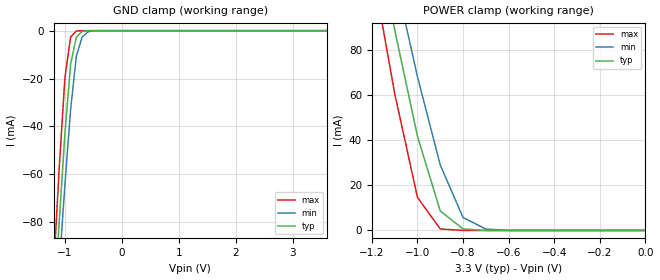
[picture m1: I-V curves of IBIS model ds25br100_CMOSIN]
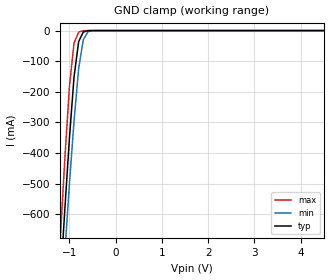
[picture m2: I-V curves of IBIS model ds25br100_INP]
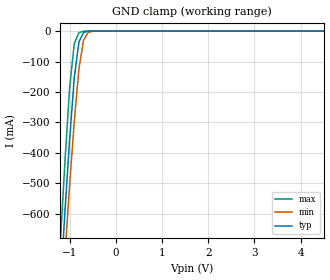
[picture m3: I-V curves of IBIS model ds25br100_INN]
|   National Semiconductor Corporation
|   IBIS Model
|   of
|   ds25br100
|  (no equalization, no pre-emphasis)
[IBIS Ver]   3.2
[Comment Char]   |_char
[File name]   ds25br100.ibs
[File Rev]   2.0
[Date]   07/17/2007
[Source]
[Notes]
Rev 1.0   Initial release - dglisic 5/30/2007
Rev 2.0   Recreated tables, verified ibis models in hspice against
   schematic simulations in spectre, updated package model
   elements.
NOTICE:   The nature of the pre-emphasis and equalization circuitry
   precludes them from being properly modeled by the simple
   I/V and V/T data in the IBIS model.  Therefore, this model
   is only valid for this device when EQ and PE pins are set
   to logic 0.
[Disclaimer]
(C) Copyright National Semiconductor Corporation 2005
   All rights reserved
   National Semiconductor Corporation hereby grants
the user of this IBIS model a non-exclusive, nontransferable
license to use this IBIS model under the following terms.
Before using this IBIS model, the user should read this
license.  If the user does not accept these terms,  the
IBIS model should be returned to National within 30 days.
   The user is granted this license only to use the
IBIS model and is not granted rights to sell, load, rent,
lease or license the IBIS model in whole or in part, or in
modified form to anyone other than user. User may modify
the IBIS model to suit its specific applications but rights
to derivative works and such modifications shall belong to
National.
   This IBIS model is provided on an "AS IS" basis and
National makes absolutely no warranty with respect to the
information contained herein.NATIONAL DISCLAIMS AND CUSTOMER
WAIVES ALL WARRANTIES, EXPRESS OR IMPLIED, INCLUDING
WARRANTIES OF MERCHANTABILITY OR FITNESS FOR A PARTICULAR
PURPOSE. The entire risk as to quality and performance is
with the Customer. ACCORDINGLY, IN NO EVENT SHALL THE
COMPANY BE LIABLE FOR ANY DAMAGES, WHETHER IN CONTRACT OR
TORT,INCLUDING ANY LOST PROFITS OR OTHER INCIDENTAL,
CONSEQUENTIAL, EXEMPLARY, OR PUNITIVE DAMAGES ARISING OUT
OF THE USE OR APPLICATION OF THE IBIS model provided in
this package.Further, National reserves the right to make
changes without notice to any product herein to improve
reliability, function, or design. National does not convey
any license under patent rights or any other intellectual
property rights, including those of third parties.
   National is not obligated to provide maintenance or support
for the licensed IBIS model.
Contact National at ATTN:INTERFACE/IBIS MODELS.
5 Foden Road, M/S 01-50, South Porltand, ME 04106
(207) 541-8467
[Copyright]
(c) Copyright 2005 National Semiconductor Corp.
[Component]   ds25br100
Si_location Pin
Timing_location Pin
[Manufacturer]   National Semiconductor Corp.
[Package]
|   TYP   MIN   MAX
R_pkg   234m   220m   256m
L_pkg   0.7041n   0.6519n   0.7785n
C_pkg   0.0612p   0.0515p   0.0707p
[Pin]   signal_name   model_name   R_pin   L_pin   C_pin
1   EQ   ds25br100_CMOSIN   243m   0.7785n  0.0533p
2   IN+   ds25br100_INP   222m   0.6629n  0.0515p
3   IN-   ds25br100_INN   221m   0.6626n  0.0516p
4   PE   ds25br100_CMOSIN   241m   0.7773n  0.0529p
5   NC   NC   NA   NA   NA
6   OUT-   ds25br100_OUTN   225m   0.6798n  0.0662p
7   OUT+   ds25br100_OUTP   220m   0.6519n  0.0517p
8   VCC   POWER   127m   0.3712n  0.0707p |double bond
[Series Pin Mapping]   pin_2   model_name
2   3   input_term
[Diff Pin] inv_pin   vdiff   tdelay_typ   tdelay_min   tdelay_max
| The '+' pin is Diff_pin and the '-' pin is the inv_pin
| Receiver Vth = +/-100mV
2   3   0.05   0   0   0
7   6   0.00   0   0   0
|   Model input termination resistor
[Model]   input_term
Model_type   Series
Polarity   Non-Inverting
C_comp   0.0pF   0.0pF   0.0pF
[Temperature Range] 25   85   -40
[Voltage Range]   3.3   3.0   3.6
| Resistance   ohm(typ)   ohm(min)   ohm(max)
[R Series]   100   85   115
| Models and submodels in the file (6): ds25br100_CMOSIN (Input), ds25br100_INP (Input), ds25br100_INN (Input), ds25br100_OUTP (Output), ds25br100_OUTN (Output), input_term (Series)
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[Model]   ds25br100_CMOSIN
Model_type Input
Polarity Non-Inverting
Vinh=2.0
Vinl=0.8
C_comp   2pF   2pF   2pF
[Model Spec]
S_overshoot_high   3.3   3.0   3.6
S_overshoot_low   0.0   0.0   0.0
[Temperature Range]   25   85   -40
[Voltage Range]   3.3   3.0   3.6
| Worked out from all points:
|   GND clamp passes 1 mA (typ) near -0.73 V on its own axis
|   POWER clamp passes 1 mA (typ) near -0.80 V on its own axis
[GND Clamp]
-3.6V     -1.151A    -1.073A    -1.257A
-1.2V     -119.2mA   -135.1mA   -100.7mA
-1.1V     -79.74mA   -98.82mA   -57.2mA
-1V       -42.96mA   -64.16mA   -19.61mA
-900mV    -13.95mA   -32.92mA   -2.641mA
-800mV    -2.76mA    -10.67mA   -143.9uA
-700mV    -354.1uA   -2.787mA   -1.241uA
-600mV    -11.59uA   -558uA     -8.6nA
-500mV    -240.8nA   -41.97uA   -83.78pA
3.6V      55.55pA    37uA       50.4pA
[POWER Clamp]
-3.6V     1.518A     1.417A     1.655A
-1.2V     141.2mA    161.6mA    117.8mA
-1.1V     89.19mA    113.7mA    60.9mA
-1V       41.87mA    68.34mA    14.7mA
-900mV    8.67mA     29.1mA     658uA
-800mV    660uA      5.729mA    7.509uA
-700mV    21.02uA    636.6uA    52.21nA
-600mV    436.7nA    37uA       420.5pA
0V        46.2pA     46.13pA    50.4pA
[Model]   ds25br100_INP
Model_type Input
Polarity Non-Inverting
Vinh=1.25
Vinl=1.15
C_comp   1.7pF   1.7pF   1.7pF
[Model Spec]
S_overshoot_high   3.3   3.0   3.6
S_overshoot_low   0.0   0.0   0.0
[Temperature Range]   25   85   -40
[Voltage Range]   3.3   3.0   3.6
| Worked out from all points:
|   GND clamp passes 1 mA (typ) near -0.62 V on its own axis
[GND Clamp]
|V(groundclamp)   I(typ)   I(min)   I(max)
-3.6V     -7.949A    -7.688A    -8.364A
-1.2V     -837.2mA   -968.2mA   -688.4mA
-1.1V     -586.8mA   -729.1mA   -422.6mA
-1V       -353.4mA   -502.6mA   -183.7mA
-900mV    -151.8mA   -295.7mA   -40.94mA
-800mV    -36.07mA   -124.3mA   -4.991mA
-700mV    -4.641mA   -29.98mA   -506.7uA
-600mV    -299.4uA   -4.1mA     -51.64uA
-500mV    -23.36uA   -273.5uA   -3.241uA
7.2V      407.9pA    9.955nA    116.1pA
[Model]   ds25br100_INN
Model_type Input
Polarity Inverting
Vinh=1.25
Vinl=1.15
C_comp   1.7pF   1.7pF   1.7pF
[Model Spec]
S_overshoot_high   3.3   3.0   3.6
S_overshoot_low   0.0   0.0   0.0
[Temperature Range]   25   85   -40
[Voltage Range]   3.3   3.0   3.6
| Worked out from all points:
|   GND clamp passes 1 mA (typ) near -0.62 V on its own axis
[GND Clamp]
|V(groundclamp)   I(typ)   I(min)   I(max)
-3.6V     -7.949A    -7.688A    -8.364A
-1.2V     -837.2mA   -968.2mA   -688.4mA
-1.1V     -586.8mA   -729.1mA   -422.6mA
-1V       -353.4mA   -502.6mA   -183.7mA
-900mV    -151.8mA   -295.7mA   -40.94mA
-800mV    -36.07mA   -124.3mA   -4.991mA
-700mV    -4.641mA   -29.98mA   -506.7uA
-600mV    -299.4uA   -4.1mA     -51.64uA
-500mV    -23.36uA   -273.5uA   -3.241uA
7.2V      407.9pA    9.955nA    116.1pA
